(* Logix 5000 AddOnInstructionDefinition export Banner_Q5X_3000_Param_v4; software revision 33.00 *)

TYPE Banner_IOL_Port_v4 :   // UDT that has all of the data items necessary to communicate with a specific Port on a IO-Link Master
STRUCT
   Port_Controlled : INT;   // Each bit represents a port on an IO-Link Master. Set to 1 to tell AOI to control that port.
   Port_Activate : INT;   // Each bit represents a port on an IO-Link Master. When ON that port will process any commands in queue.
   Port_Read : INT;   // Each bit represents a port on an IO-Link Master. Used to determine when device AOI has requested a Read command.
   Port_Write : INT;   // Each bit represents a port on an IO-Link Master. Used to determine when device AOI has requested a Write command.
   Port_RW_Complete : INT;   // Each bit represents a port on an IO-Link Master. Tells device AOI that Read or Write request has been completed.
   Port_Device_Read : INT;
   Data_Transfer : SINT[190];   // Array to transfer data from IO-Master to device AOIs.
END_STRUCT
END_TYPE

TYPE Banner_Q5X_3000_RD_v4 :   // UDT that stores the Write Data for a Q5X TOF.
STRUCT
   Master_Cycle_Time : INT;
   Min_Cycle_Time : INT;
   M_Sequence_Capability : INT;
   IO_Link_Version_ID : INT;
   Process_Data_Input_Length : INT;
   Process_Data_Output_Length : INT;
   Combined_Vendor_ID : DINT;   // IO-Link Vendor ID
   Vendor_ID1 : INT;
   Vendor_ID2 : INT;
   Combined_Device_ID : DINT;   // IO-Link Device ID
   Device_ID1 : INT;
   Device_ID2 : INT;
   Device_ID3 : INT;
   Serial_Number : STRING;
   Teach_State : SINT;
   SP1_TP1 : SINT;
   SP1_TP2 : SINT;
   Measurement_1 : DINT;
   Excess_Gain : DINT;   // Amount of singla measured over the minimum threshold.
   Stability : SINT;
   Multiple_Peak_State : SINT;   // 0 = Multiple peaks not present, 1 = Multiple peaks present
   Emitter_Status : SINT;   // 0 = Active, 1 = Inactive
   Laser_Fault_Status : SINT;   // 0 = No Fault, 1 = Fault Present
   BDC1_Totalizer_Counts : DINT;
   Analog_Value : DINT;   // Output Analog value.
   Last_Taught_Temperature : DINT;   // Internal Temperature the last time device was taught.
   All_Time_Run_Time : DINT;   // Read only counter that tracks the total time sensor has been running since manufacture. Value in Hours.
   Display : STRING;   // Last Display information
   MDC_Lower_Limit : DINT;
   MDC_Upper_Limit : DINT;
   MDC_Unit : INT;
   MDC_Scale : SINT;
END_STRUCT
END_TYPE

TYPE Banner_Q5X_3000_v4 :   // All of the parameters for a Q5X Analog.
STRUCT
   Initial_Global_Read : BOOL;   // Determines if all of the IO-Link data has been read into the PLC yet
   Command : INT;   // Value placed in here will activate a read or write to a specifc IO-Link Index
   Read_Data : Banner_Q5X_3000_RD_v4;   // Read Only Data
   Write_Data : Banner_Q5X_3000_WD_v4;   // Write Data
   Archive : Banner_Q5X_3000_WD_v4;   // Archive Data
   Reset : BOOL;   // Resets AOI. This will force a complete parameter read of the sensor.
END_STRUCT
END_TYPE

TYPE Banner_Q5X_3000_WD_v4 :   // UDT that stores the Write Data for a Q5X Analog.
STRUCT
   System_Command : INT;   // See IODD file for list of commands that can be activated via the System Command interface
   Parameter_Access_Lock : SINT;   // Write access to all parameters is prohibited while value is 1. Only this parameter can be adjusted when value is 1.
   Data_Storage_Lock : SINT;   // Automatic data storage is disabled when this value is equal to 1. Read access is not affected.
   Local_Parameterization_Lock : SINT;   // Parameterization via local control elements on device is disabled.
   Local_User_Interface_Lock : SINT;   // Operation of local user interface is disabled.
   Teach_in_Channel : SINT;   // 0 = Default, 1 = BDC1, 2 = BDC2
   BDC1_Setpoint_1 : DINT;
   BDC1_Setpoint_2 : DINT;   // In FGS, defines the second switching point. Other modes do not use this parameter.
   BDC1_Switchpoint_Logic : INT;   // 0 = Light Operate, 1 = Dark Operate
   BDC1_Mode : INT;   // 1 = 1Pt BGS, 128 = 2Pt Static BGS, 129 = Dynamic BGS, 130 = 1Pt Window (FGS), 131 = Dual Teach
   BDC1_Hysteresis : INT;   // Hysteresis value for the switchpoint. A value of 0 will result in automatically calculated hysteresis
   Response_Speed : SINT;   // 0 = Speed 0, 1 = Speed 1, 2 = Speed 2, 3 = Speed 3
   Secondary_Output_Mode : SINT;   // 0 = Independent Output, 1 = Complementary Output, 2 = Pulse Frequency Output
   Zero_Reference_Location : SINT;   // 0 = Near, 1 = Far
   Shift_Zero_after_Teach : SINT;   // 0 = Off, 1 = On
   Display_Read : SINT;   // 0 = On, 1 = On Inverted, 2 = Off, 3 = Off Inverted
   Display_Units : SINT;   // 0 = Centimeters, 1 = Inches, 2 = Millimeters
   Pushbutton_Lockout : SINT;   // 0 = No Lockout, 1 = Pushbuttons Locked, 2 = Operator Lockout
   Output_Polarity : SINT;   // 0 = Default, 1 = PNP, 2 = NPN
   IOL_Filter_Time : INT;   // Time to average IOl process data measurement between updates
   Include_Binary : SINT;   // 0 = Include, 1 = Don't Include, 2= Measurement Device
   Measurement_1 : SINT;   // 0 = Disabled, 1 = Excess Gain, 2 = Excess Gain / 10, 3 = Channel 1 Dual Mode Percent
   Measurement_2 : SINT;   // 0 = Disabled, 1 = Distance Value, 2 = Displayed Distance, 3 = Channel 2 Dual Mode Percent
   BDC1_Delay_Mode : SINT;   // 0 = Disabled, 1 = On Off Delay, 2 = Oneshot, 3 = Totalizer
   BDC1_Delay_Timer_1 : DINT;   // 0 to 90000
   BDC1_Delay_Timer_2 : DINT;   // 0 to 90000
   BDC1_BGS_Teach_Offset : SINT;   // 0 = Auto, 1 = User Selected
   BDC1_FGS_Window_Size : SINT;   // 0 = Auto, 1 = User Selected
   BDC1_User_Teach_Offset : DINT;   // Mode must be FGS of BGS. Set the user defined offset. Can be positive or negative.
   BDC1_User_FGS_Window_Size : DINT;   // Mode must be FGS. Set the +/- window value.
   BDC1_Auto_Thresholding : SINT;   // 0 = On, 1 = Off, 2 = High Speed
   Resettable_Run_Time : DINT;
   AO1_Setpoint_SP1 : DINT;
   AO1_Setpoint_SP2 : DINT;
   AO1_Output_Type : SINT;   // 0 = 4-20mA, 1 = 0-10V
   AO1_Teach_Selection : SINT;   // 0 = 2-point, 1 = 1-point
   AO1_Slope : SINT;
   AO1_Loss_of_Signal : SINT;   // 0 = positive, 1 = negative
   AO1_Midpoint_Teach_Offset_Size : DINT;
   AO1_Trigger : SINT;   // 0 = Trigger Sample, 1 = Trigger Average, 2 = Trigger Max, 3 = Trigger Min, 4 = Trigger Range, 5 = Trigger Track Max, 6 = Trigger Track Min
   AO1_Average : SINT;
   All_Time_Run_Time_Event_Time : DINT;
   Resettable_Run_Time_Event_Time : DINT;
END_STRUCT
END_TYPE

ADD_ON_INSTRUCTION Banner_Q5X_3000_Param_v4   (* revision 4.1, vendor Banner Engineering *)
// AOI to read and write parameter data to an IO-Link Q5X 3000 Analog.
VAR_IN_OUT
   Q5X : Banner_Q5X_3000_v4; {required}
   Port_Data : Banner_IOL_Port_v4; {required}
END_VAR
VAR_INPUT
   Port : DINT; {required}
END_VAR
VAR
   Local_Control : DINT; {access None}
   Global_Read_Command_Value : INT; {access None}
   Global_Write_Command_Value : INT; {access None}
   Command_Being_Processed : BOOL; {access None}
   Update_Archive : BOOL; {access None}
   Index_Write_Inprocess : INT; {access None}
   Index_Write_Control : INT; {access None}
   Inprocess_Index : DINT; {access None}
END_VAR

ROUTINE Logic   (* ladder *)
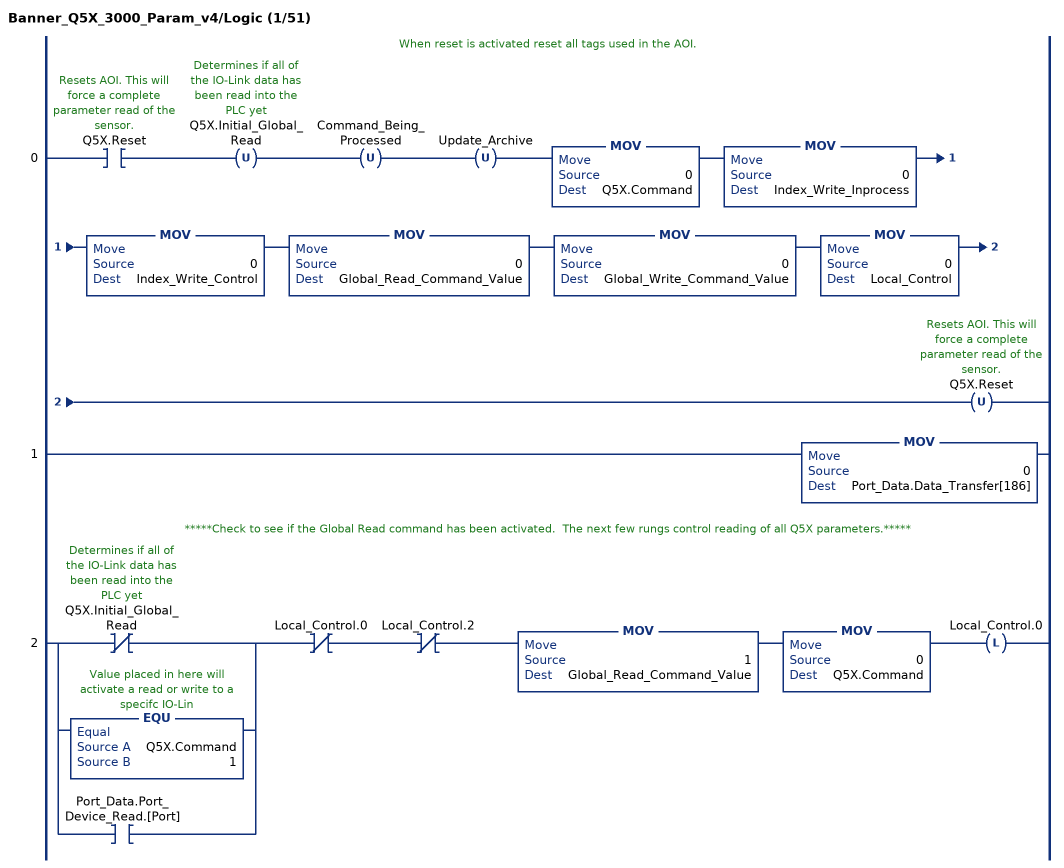
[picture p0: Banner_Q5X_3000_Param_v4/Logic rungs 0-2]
   // When reset is activated reset all tags used in the AOI.
   0: XIC(Q5X.Reset)OTU(Q5X.Initial_Global_Read)OTU(Command_Being_Processed)OTU(Update_Archive)MOV(0,Q5X.Command)MOV(0,Index_Write_Inprocess)MOV(0,Index_Write_Control)MOV(0,Global_Read_Command_Value)MOV(0,Global_Write_Command_Value)MOV(0,Local_Control)OTU(Q5X.Reset);
   1: MOV(0,Port_Data.Data_Transfer[186]);
   // *****Check to see if the Global Read command has been activated.  The next few rungs control reading of all Q5X parameters.*****
   2: [XIO(Q5X.Initial_Global_Read) ,EQU(Q5X.Command,1) ,XIC(Port_Data.Port_Device_Read.[Port]) ]XIO(Local_Control.0)XIO(Local_Control.2)MOV(1,Global_Read_Command_Value)MOV(0,Q5X.Command)OTL(Local_Control.0);
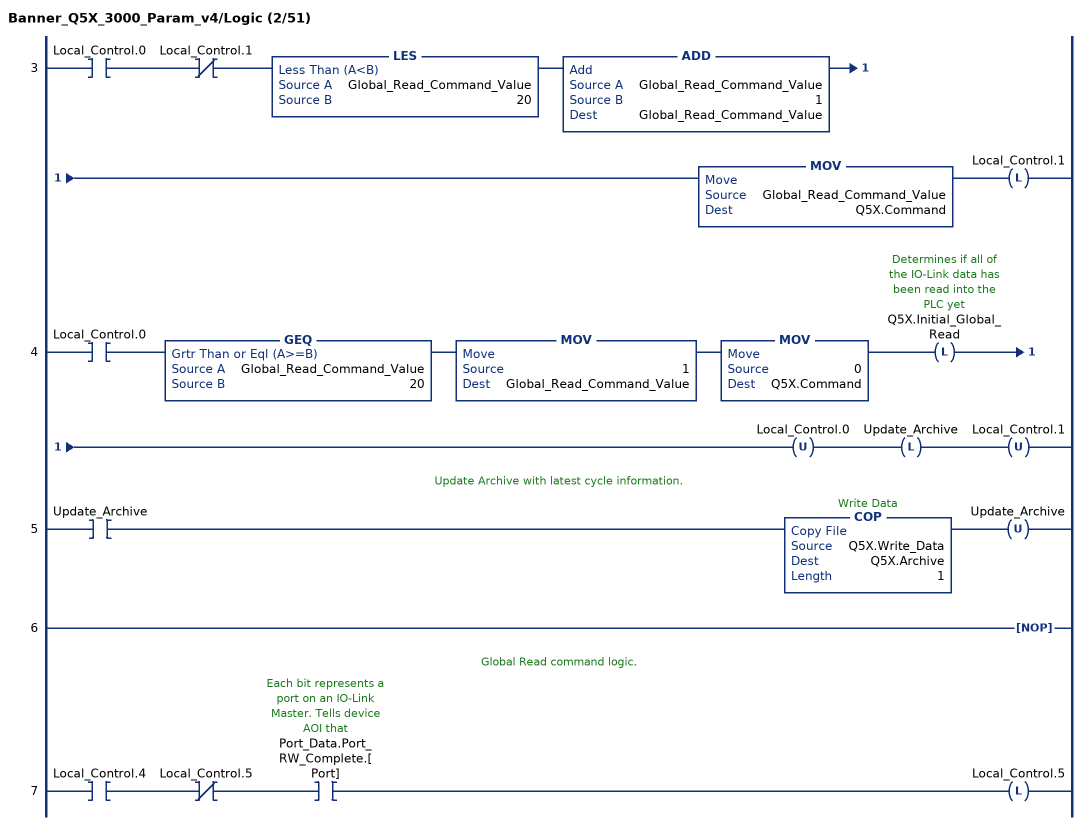
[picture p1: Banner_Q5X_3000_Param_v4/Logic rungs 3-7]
   3: XIC(Local_Control.0)XIO(Local_Control.1)LES(Global_Read_Command_Value,20)ADD(Global_Read_Command_Value,1,Global_Read_Command_Value)MOV(Global_Read_Command_Value,Q5X.Command)OTL(Local_Control.1);
   4: XIC(Local_Control.0)GEQ(Global_Read_Command_Value,20)MOV(1,Global_Read_Command_Value)MOV(0,Q5X.Command)OTL(Q5X.Initial_Global_Read)OTU(Local_Control.0)OTL(Update_Archive)OTU(Local_Control.1);
   // Update Archive with latest cycle information.
   5: XIC(Update_Archive)COP(Q5X.Write_Data,Q5X.Archive,1)OTU(Update_Archive);
   6: NOP();
   // Global Read command logic.
   7: XIC(Local_Control.4)XIO(Local_Control.5)XIC(Port_Data.Port_RW_Complete.[Port])OTL(Local_Control.5);
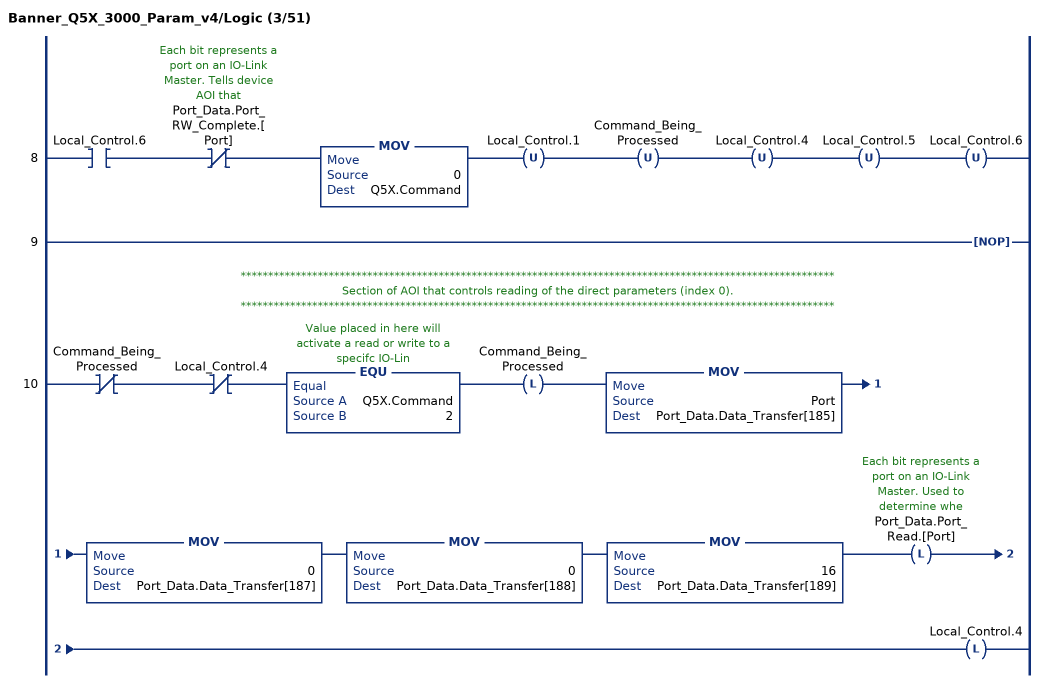
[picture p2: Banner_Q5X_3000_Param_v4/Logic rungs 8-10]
   8: XIC(Local_Control.6)XIO(Port_Data.Port_RW_Complete.[Port])MOV(0,Q5X.Command)OTU(Local_Control.1)OTU(Command_Being_Processed)OTU(Local_Control.4)OTU(Local_Control.5)OTU(Local_Control.6);
   9: NOP();
   // ************************************************************************************************************
   // Section of AOI that controls reading of the direct parameters (index 0).
   // ************************************************************************************************************
   10: XIO(Command_Being_Processed)XIO(Local_Control.4)EQU(Q5X.Command,2)OTL(Command_Being_Processed)MOV(Port,Port_Data.Data_Transfer[185])MOV(0,Port_Data.Data_Transfer[187])MOV(0,Port_Data.Data_Transfer[188])MOV(16,Port_Data.Data_Transfer[189])OTL(Port_Data.Port_Read.[Port])OTL(Local_Control.4);
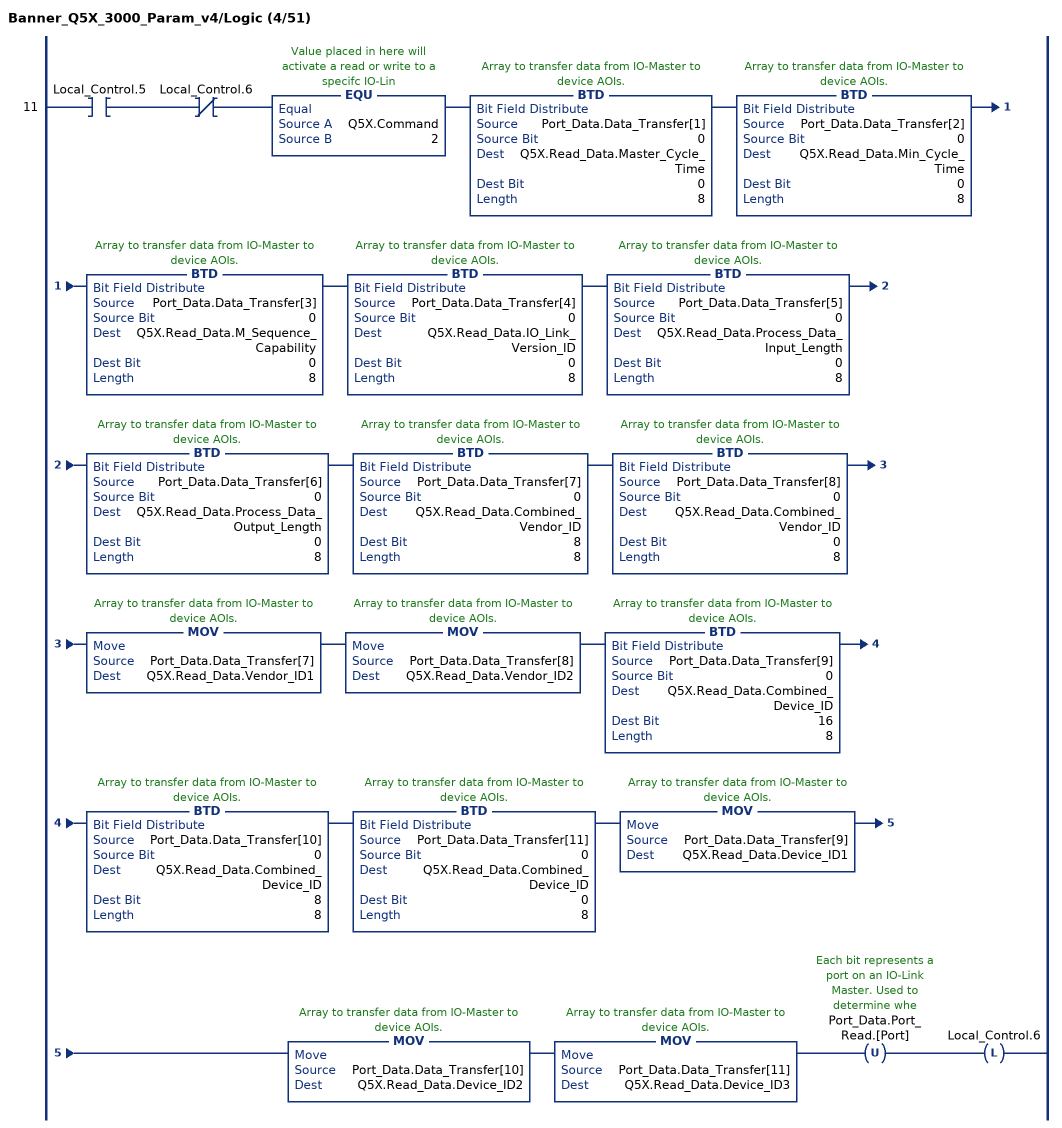
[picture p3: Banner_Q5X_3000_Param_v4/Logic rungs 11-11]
   11: XIC(Local_Control.5)XIO(Local_Control.6)EQU(Q5X.Command,2)BTD(Port_Data.Data_Transfer[1],0,Q5X.Read_Data.Master_Cycle_Time,0,8)BTD(Port_Data.Data_Transfer[2],0,Q5X.Read_Data.Min_Cycle_Time,0,8)BTD(Port_Data.Data_Transfer[3],0,Q5X.Read_Data.M_Sequence_Capability,0,8)BTD(Port_Data.Data_Transfer[4],0,Q5X.Read_Data.IO_Link_Version_ID,0,8)BTD(Port_Data.Data_Transfer[5],0,Q5X.Read_Data.Process_Data_Input_Length,0,8)BTD(Port_Data.Data_Transfer[6],0,Q5X.Read_Data.Process_Data_Output_Length,0,8)BTD(Port_Data.Data_Transfer[7],0,Q5X.Read_Data.Combined_Vendor_ID,8,8)BTD(Port_Data.Data_Transfer[8],0,Q5X.Read_Data.Combined_Vendor_ID,0,8)MOV(Port_Data.Data_Transfer[7],Q5X.Read_Data.Vendor_ID1)MOV(Port_Data.Data_Transfer[8],Q5X.Read_Data.Vendor_ID2)BTD(Port_Data.Data_Transfer[9],0,Q5X.Read_Data.Combined_Device_ID,16,8)BTD(Port_Data.Data_Transfer[10],0,Q5X.Read_Data.Combined_Device_ID,8,8)BTD(Port_Data.Data_Transfer[11],0,Q5X.Read_Data.Combined_Device_ID,0,8)MOV(Port_Data.Data_Transfer[9],Q5X.Read_Data.Device_ID1)MOV(Port_Data.Data_Transfer[10],Q5X.Read_Data.Device_ID2)MOV(Port_Data.Data_Transfer[11],Q5X.Read_Data.Device_ID3)OTU(Port_Data.Port_Read.[Port])OTL(Local_Control.6);
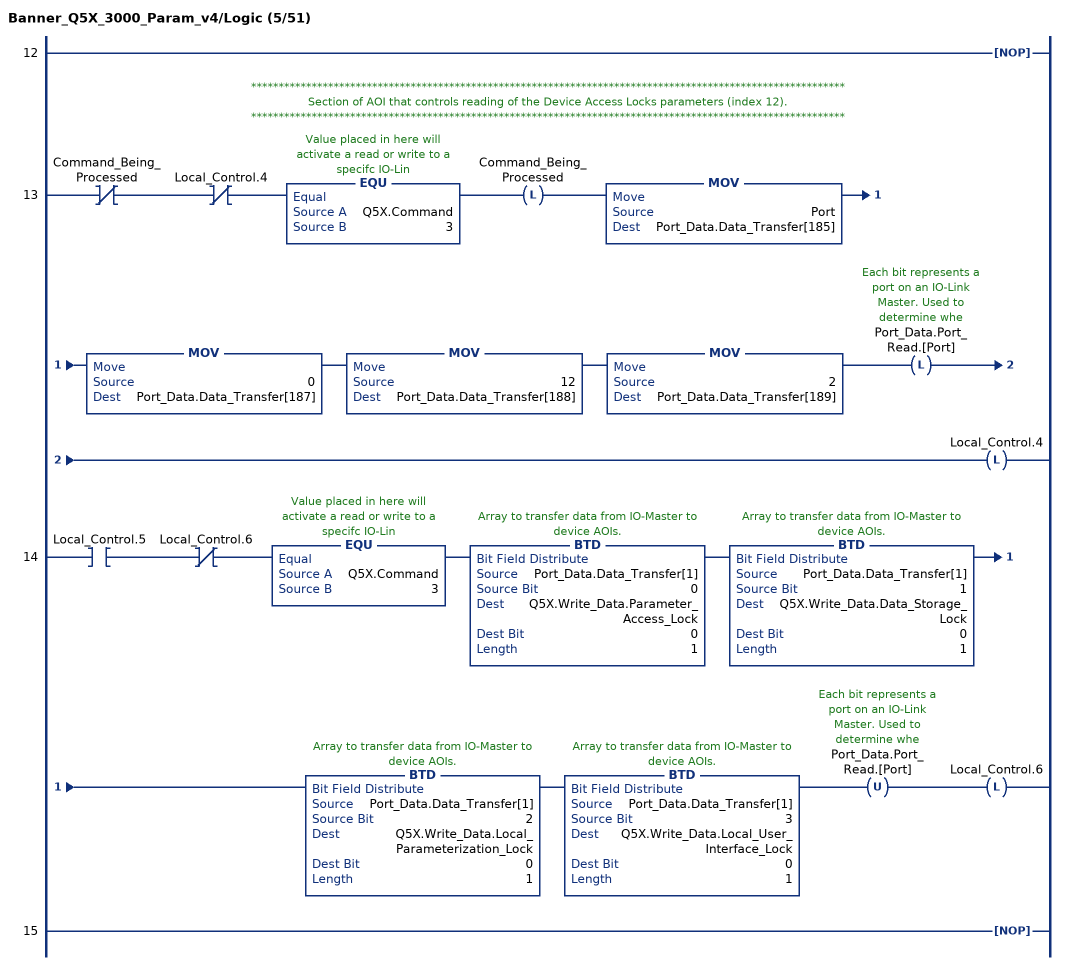
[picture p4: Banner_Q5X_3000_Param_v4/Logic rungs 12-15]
   12: NOP();
   // ************************************************************************************************************
   // Section of AOI that controls reading of the Device Access Locks parameters (index 12).
   // ************************************************************************************************************
   13: XIO(Command_Being_Processed)XIO(Local_Control.4)EQU(Q5X.Command,3)OTL(Command_Being_Processed)MOV(Port,Port_Data.Data_Transfer[185])MOV(0,Port_Data.Data_Transfer[187])MOV(12,Port_Data.Data_Transfer[188])MOV(2,Port_Data.Data_Transfer[189])OTL(Port_Data.Port_Read.[Port])OTL(Local_Control.4);
   14: XIC(Local_Control.5)XIO(Local_Control.6)EQU(Q5X.Command,3)BTD(Port_Data.Data_Transfer[1],0,Q5X.Write_Data.Parameter_Access_Lock,0,1)BTD(Port_Data.Data_Transfer[1],1,Q5X.Write_Data.Data_Storage_Lock,0,1)BTD(Port_Data.Data_Transfer[1],2,Q5X.Write_Data.Local_Parameterization_Lock,0,1)BTD(Port_Data.Data_Transfer[1],3,Q5X.Write_Data.Local_User_Interface_Lock,0,1)OTU(Port_Data.Port_Read.[Port])OTL(Local_Control.6);
   15: NOP();
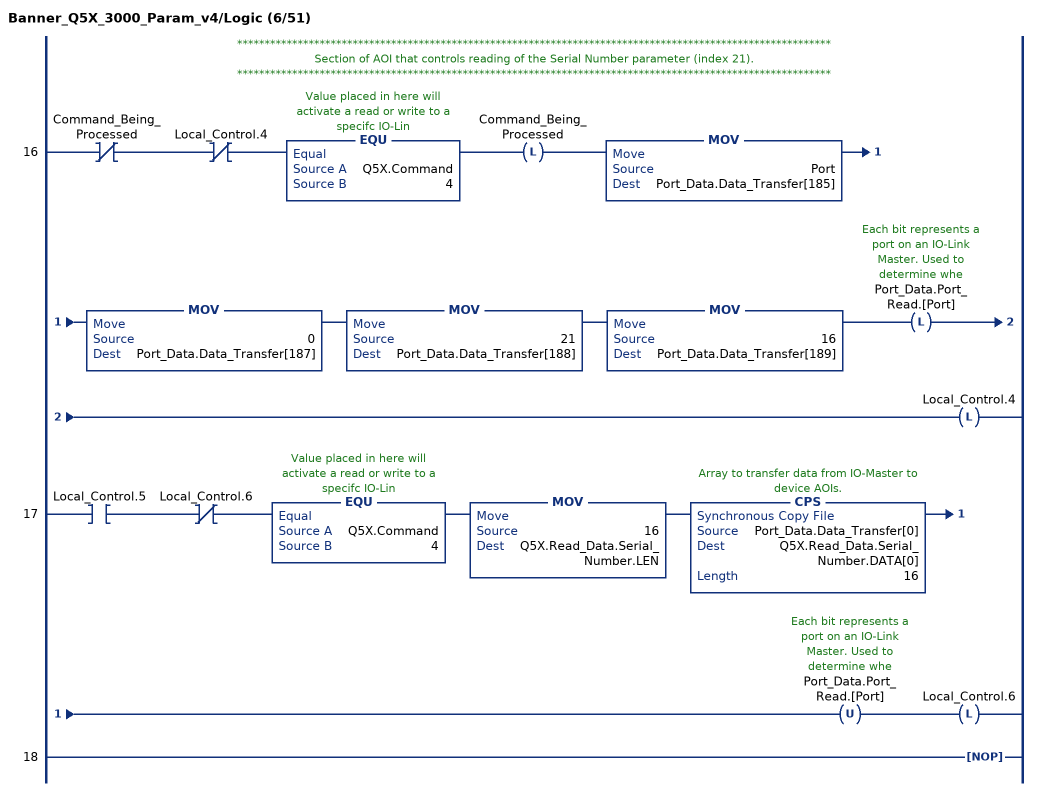
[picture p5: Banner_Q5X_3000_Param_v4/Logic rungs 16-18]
   // ************************************************************************************************************
   // Section of AOI that controls reading of the Serial Number parameter (index 21).
   // ************************************************************************************************************
   16: XIO(Command_Being_Processed)XIO(Local_Control.4)EQU(Q5X.Command,4)OTL(Command_Being_Processed)MOV(Port,Port_Data.Data_Transfer[185])MOV(0,Port_Data.Data_Transfer[187])MOV(21,Port_Data.Data_Transfer[188])MOV(16,Port_Data.Data_Transfer[189])OTL(Port_Data.Port_Read.[Port])OTL(Local_Control.4);
   17: XIC(Local_Control.5)XIO(Local_Control.6)EQU(Q5X.Command,4)MOV(16,Q5X.Read_Data.Serial_Number.LEN)CPS(Port_Data.Data_Transfer[0],Q5X.Read_Data.Serial_Number.DATA[0],16)OTU(Port_Data.Port_Read.[Port])OTL(Local_Control.6);
   18: NOP();
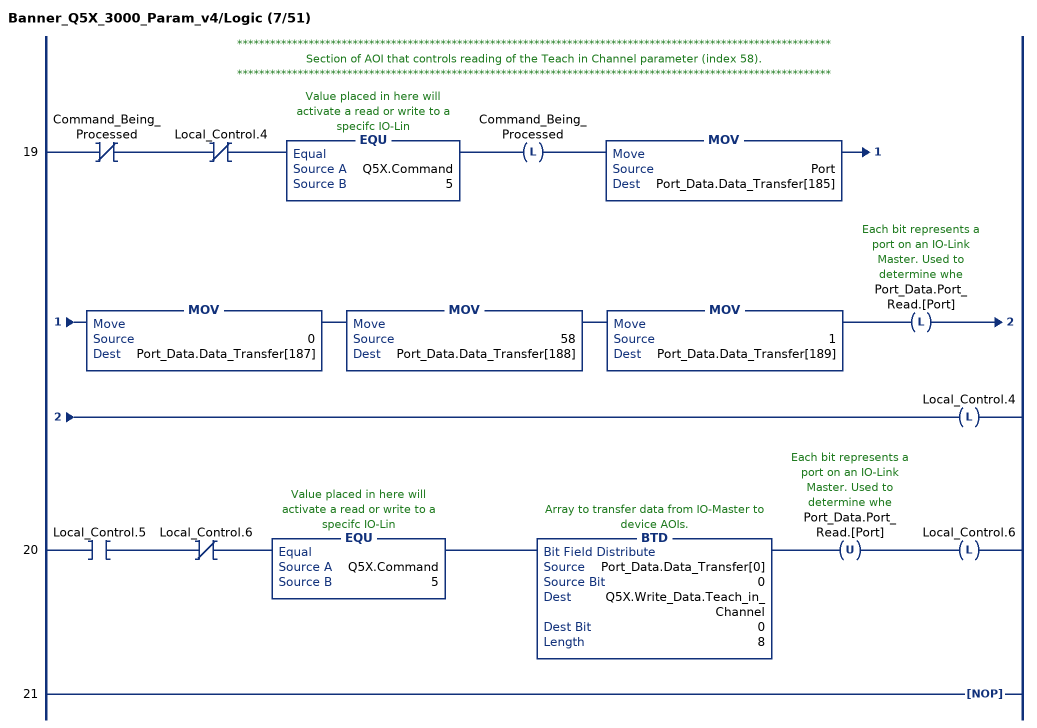
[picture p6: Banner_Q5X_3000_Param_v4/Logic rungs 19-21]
   // ************************************************************************************************************
   // Section of AOI that controls reading of the Teach in Channel parameter (index 58).
   // ************************************************************************************************************
   19: XIO(Command_Being_Processed)XIO(Local_Control.4)EQU(Q5X.Command,5)OTL(Command_Being_Processed)MOV(Port,Port_Data.Data_Transfer[185])MOV(0,Port_Data.Data_Transfer[187])MOV(58,Port_Data.Data_Transfer[188])MOV(1,Port_Data.Data_Transfer[189])OTL(Port_Data.Port_Read.[Port])OTL(Local_Control.4);
   20: XIC(Local_Control.5)XIO(Local_Control.6)EQU(Q5X.Command,5)BTD(Port_Data.Data_Transfer[0],0,Q5X.Write_Data.Teach_in_Channel,0,8)OTU(Port_Data.Port_Read.[Port])OTL(Local_Control.6);
   21: NOP();
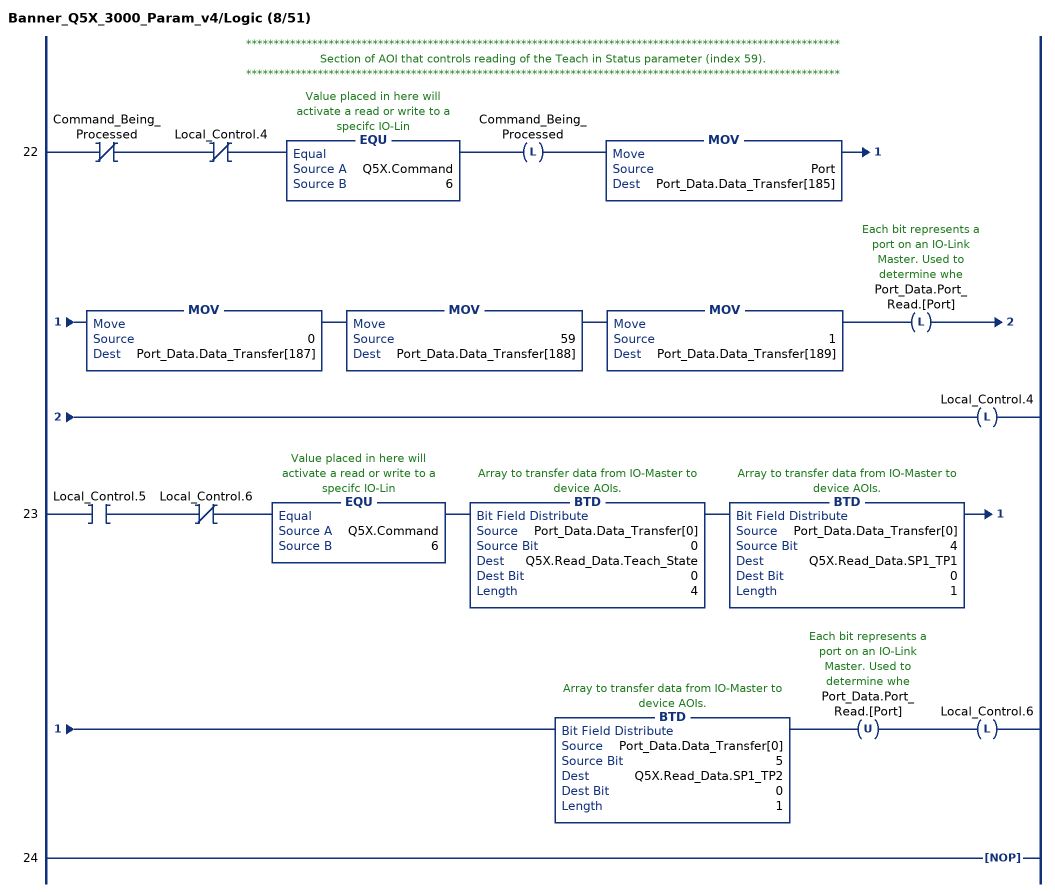
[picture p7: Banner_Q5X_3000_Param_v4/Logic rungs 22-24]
   // ************************************************************************************************************
   // Section of AOI that controls reading of the Teach in Status parameter (index 59).
   // ************************************************************************************************************
   22: XIO(Command_Being_Processed)XIO(Local_Control.4)EQU(Q5X.Command,6)OTL(Command_Being_Processed)MOV(Port,Port_Data.Data_Transfer[185])MOV(0,Port_Data.Data_Transfer[187])MOV(59,Port_Data.Data_Transfer[188])MOV(1,Port_Data.Data_Transfer[189])OTL(Port_Data.Port_Read.[Port])OTL(Local_Control.4);
   23: XIC(Local_Control.5)XIO(Local_Control.6)EQU(Q5X.Command,6)BTD(Port_Data.Data_Transfer[0],0,Q5X.Read_Data.Teach_State,0,4)BTD(Port_Data.Data_Transfer[0],4,Q5X.Read_Data.SP1_TP1,0,1)BTD(Port_Data.Data_Transfer[0],5,Q5X.Read_Data.SP1_TP2,0,1)OTU(Port_Data.Port_Read.[Port])OTL(Local_Control.6);
   24: NOP();
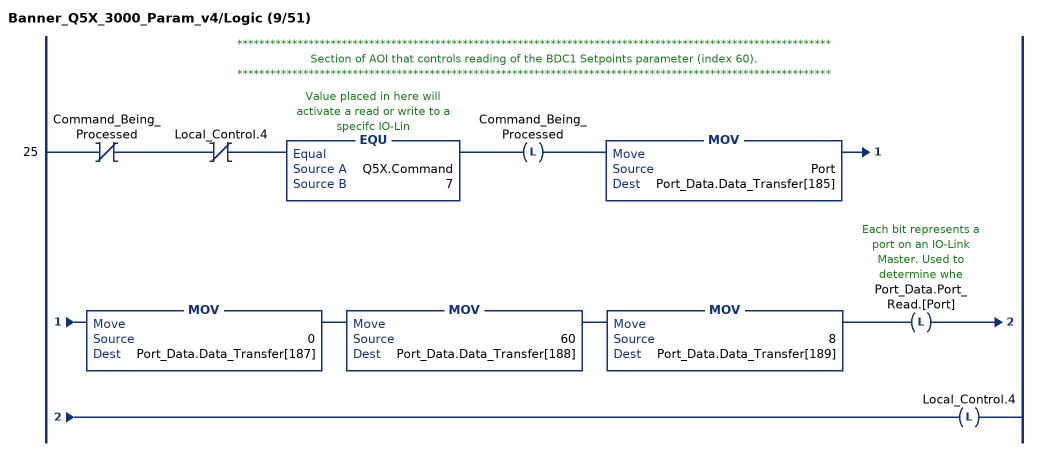
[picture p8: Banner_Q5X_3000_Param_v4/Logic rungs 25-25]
   // ************************************************************************************************************
   // Section of AOI that controls reading of the BDC1 Setpoints parameter (index 60).
   // ************************************************************************************************************
   25: XIO(Command_Being_Processed)XIO(Local_Control.4)EQU(Q5X.Command,7)OTL(Command_Being_Processed)MOV(Port,Port_Data.Data_Transfer[185])MOV(0,Port_Data.Data_Transfer[187])MOV(60,Port_Data.Data_Transfer[188])MOV(8,Port_Data.Data_Transfer[189])OTL(Port_Data.Port_Read.[Port])OTL(Local_Control.4);
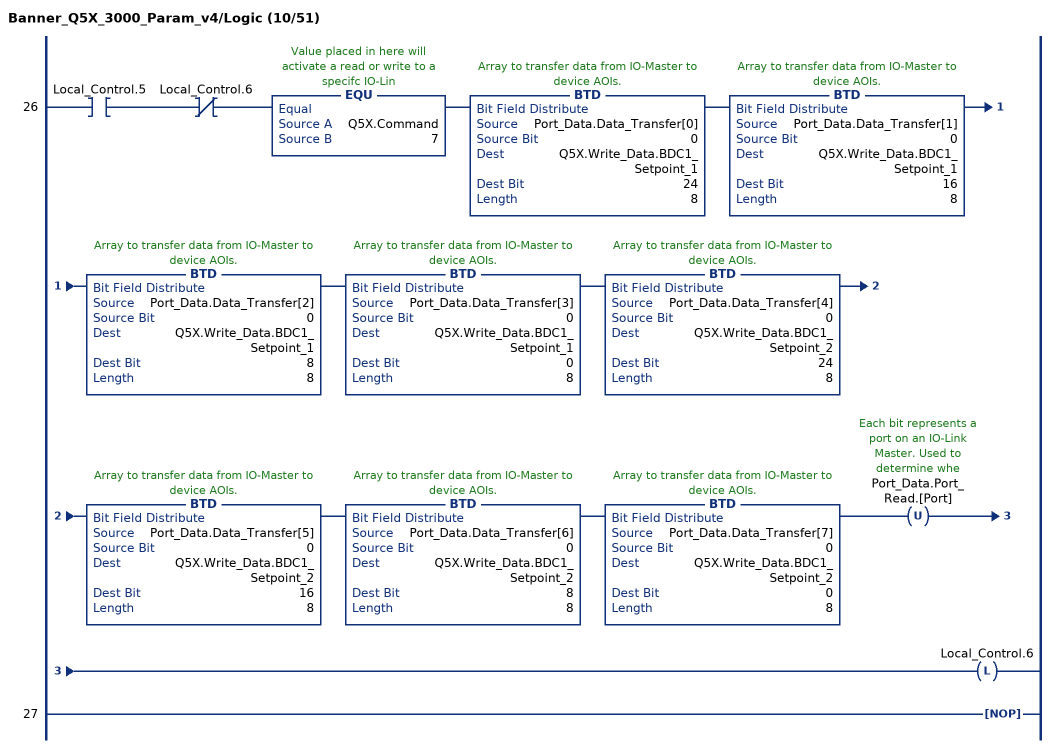
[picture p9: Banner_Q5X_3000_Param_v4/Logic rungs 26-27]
   26: XIC(Local_Control.5)XIO(Local_Control.6)EQU(Q5X.Command,7)BTD(Port_Data.Data_Transfer[0],0,Q5X.Write_Data.BDC1_Setpoint_1,24,8)BTD(Port_Data.Data_Transfer[1],0,Q5X.Write_Data.BDC1_Setpoint_1,16,8)BTD(Port_Data.Data_Transfer[2],0,Q5X.Write_Data.BDC1_Setpoint_1,8,8)BTD(Port_Data.Data_Transfer[3],0,Q5X.Write_Data.BDC1_Setpoint_1,0,8)BTD(Port_Data.Data_Transfer[4],0,Q5X.Write_Data.BDC1_Setpoint_2,24,8)BTD(Port_Data.Data_Transfer[5],0,Q5X.Write_Data.BDC1_Setpoint_2,16,8)BTD(Port_Data.Data_Transfer[6],0,Q5X.Write_Data.BDC1_Setpoint_2,8,8)BTD(Port_Data.Data_Transfer[7],0,Q5X.Write_Data.BDC1_Setpoint_2,0,8)OTU(Port_Data.Port_Read.[Port])OTL(Local_Control.6);
   27: NOP();
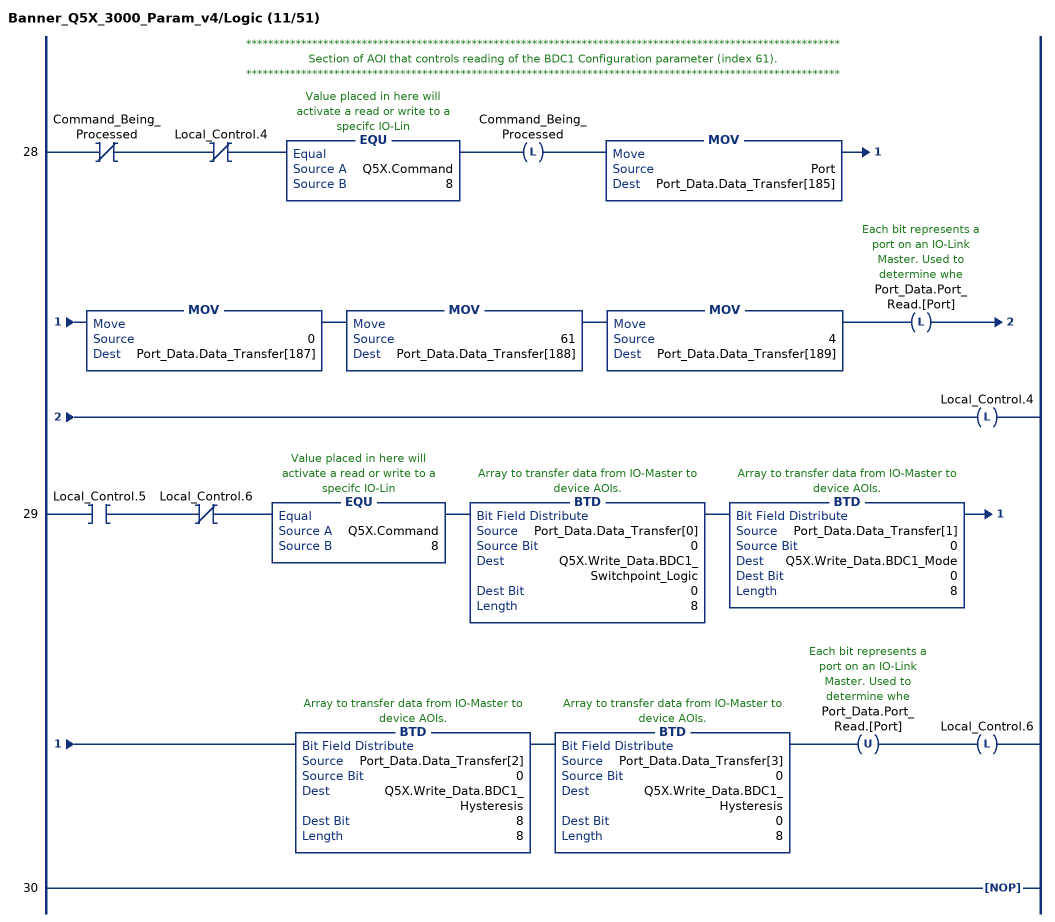
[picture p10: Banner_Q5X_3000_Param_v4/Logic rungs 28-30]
   // ************************************************************************************************************
   // Section of AOI that controls reading of the BDC1 Configuration parameter (index 61).
   // ************************************************************************************************************
   28: XIO(Command_Being_Processed)XIO(Local_Control.4)EQU(Q5X.Command,8)OTL(Command_Being_Processed)MOV(Port,Port_Data.Data_Transfer[185])MOV(0,Port_Data.Data_Transfer[187])MOV(61,Port_Data.Data_Transfer[188])MOV(4,Port_Data.Data_Transfer[189])OTL(Port_Data.Port_Read.[Port])OTL(Local_Control.4);
   29: XIC(Local_Control.5)XIO(Local_Control.6)EQU(Q5X.Command,8)BTD(Port_Data.Data_Transfer[0],0,Q5X.Write_Data.BDC1_Switchpoint_Logic,0,8)BTD(Port_Data.Data_Transfer[1],0,Q5X.Write_Data.BDC1_Mode,0,8)BTD(Port_Data.Data_Transfer[2],0,Q5X.Write_Data.BDC1_Hysteresis,8,8)BTD(Port_Data.Data_Transfer[3],0,Q5X.Write_Data.BDC1_Hysteresis,0,8)OTU(Port_Data.Port_Read.[Port])OTL(Local_Control.6);
   30: NOP();
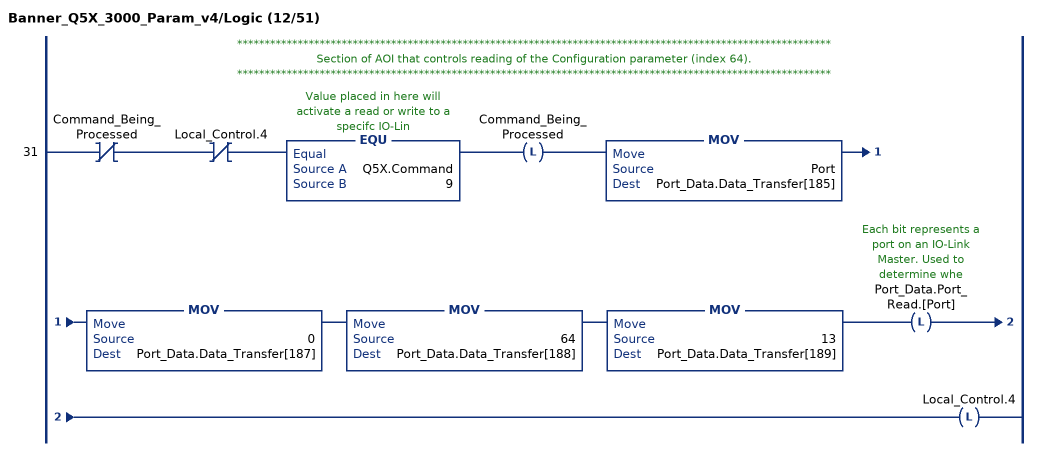
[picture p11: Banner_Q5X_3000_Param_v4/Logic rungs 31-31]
   // ************************************************************************************************************
   // Section of AOI that controls reading of the Configuration parameter (index 64).
   // ************************************************************************************************************
   31: XIO(Command_Being_Processed)XIO(Local_Control.4)EQU(Q5X.Command,9)OTL(Command_Being_Processed)MOV(Port,Port_Data.Data_Transfer[185])MOV(0,Port_Data.Data_Transfer[187])MOV(64,Port_Data.Data_Transfer[188])MOV(13,Port_Data.Data_Transfer[189])OTL(Port_Data.Port_Read.[Port])OTL(Local_Control.4);
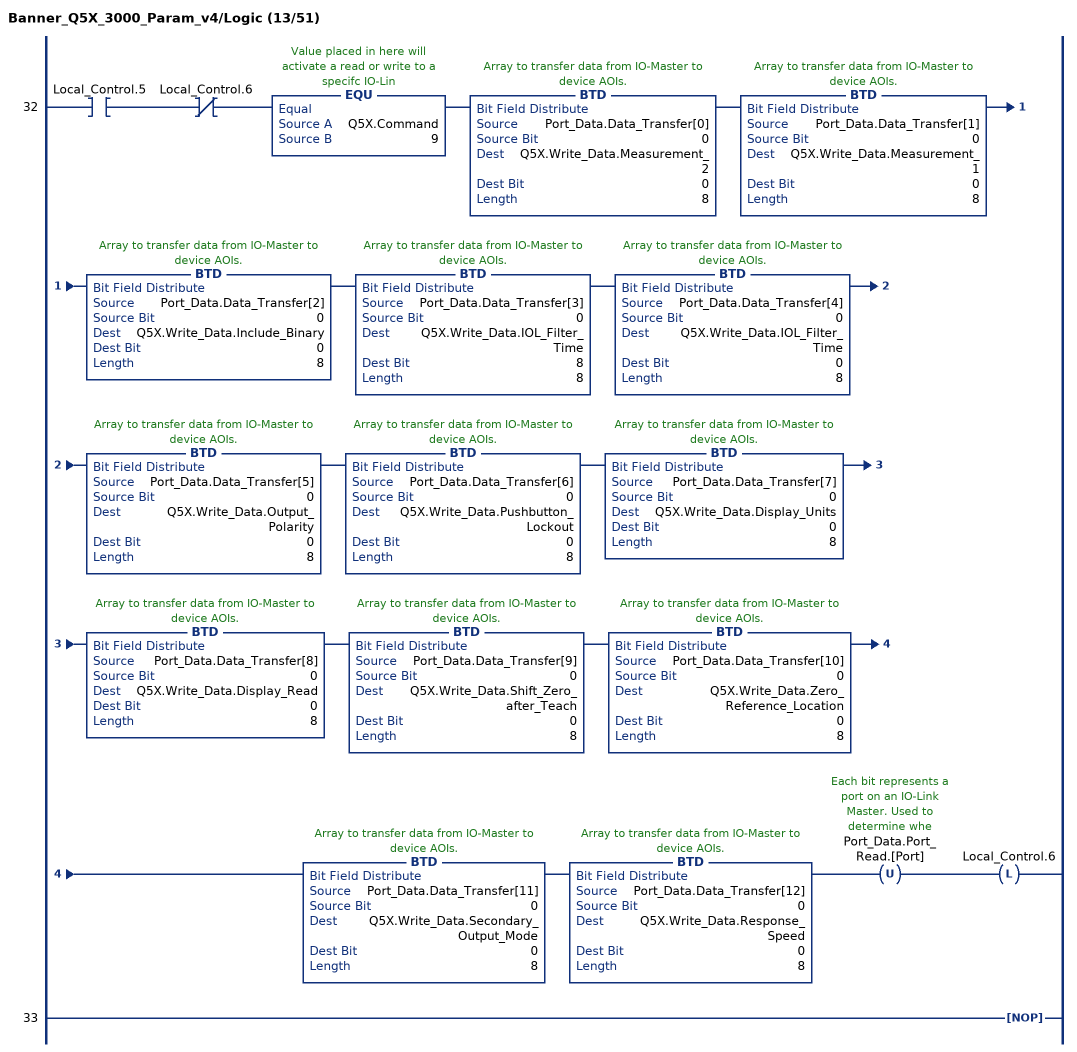
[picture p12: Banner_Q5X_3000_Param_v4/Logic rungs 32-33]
   32: XIC(Local_Control.5)XIO(Local_Control.6)EQU(Q5X.Command,9)BTD(Port_Data.Data_Transfer[0],0,Q5X.Write_Data.Measurement_2,0,8)BTD(Port_Data.Data_Transfer[1],0,Q5X.Write_Data.Measurement_1,0,8)BTD(Port_Data.Data_Transfer[2],0,Q5X.Write_Data.Include_Binary,0,8)BTD(Port_Data.Data_Transfer[3],0,Q5X.Write_Data.IOL_Filter_Time,8,8)BTD(Port_Data.Data_Transfer[4],0,Q5X.Write_Data.IOL_Filter_Time,0,8)BTD(Port_Data.Data_Transfer[5],0,Q5X.Write_Data.Output_Polarity,0,8)BTD(Port_Data.Data_Transfer[6],0,Q5X.Write_Data.Pushbutton_Lockout,0,8)BTD(Port_Data.Data_Transfer[7],0,Q5X.Write_Data.Display_Units,0,8)BTD(Port_Data.Data_Transfer[8],0,Q5X.Write_Data.Display_Read,0,8)BTD(Port_Data.Data_Transfer[9],0,Q5X.Write_Data.Shift_Zero_after_Teach,0,8)BTD(Port_Data.Data_Transfer[10],0,Q5X.Write_Data.Zero_Reference_Location,0,8)BTD(Port_Data.Data_Transfer[11],0,Q5X.Write_Data.Secondary_Output_Mode,0,8)BTD(Port_Data.Data_Transfer[12],0,Q5X.Write_Data.Response_Speed,0,8)OTU(Port_Data.Port_Read.[Port])OTL(Local_Control.6);
   33: NOP();
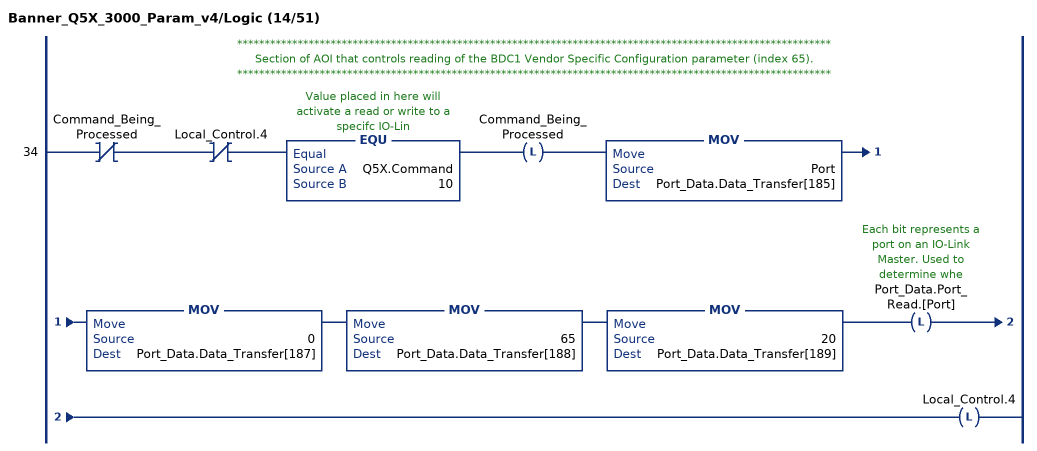
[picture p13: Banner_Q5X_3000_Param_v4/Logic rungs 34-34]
   // ************************************************************************************************************
   // Section of AOI that controls reading of the BDC1 Vendor Specific Configuration parameter (index 65).
   // ************************************************************************************************************
   34: XIO(Command_Being_Processed)XIO(Local_Control.4)EQU(Q5X.Command,10)OTL(Command_Being_Processed)MOV(Port,Port_Data.Data_Transfer[185])MOV(0,Port_Data.Data_Transfer[187])MOV(65,Port_Data.Data_Transfer[188])MOV(20,Port_Data.Data_Transfer[189])OTL(Port_Data.Port_Read.[Port])OTL(Local_Control.4);
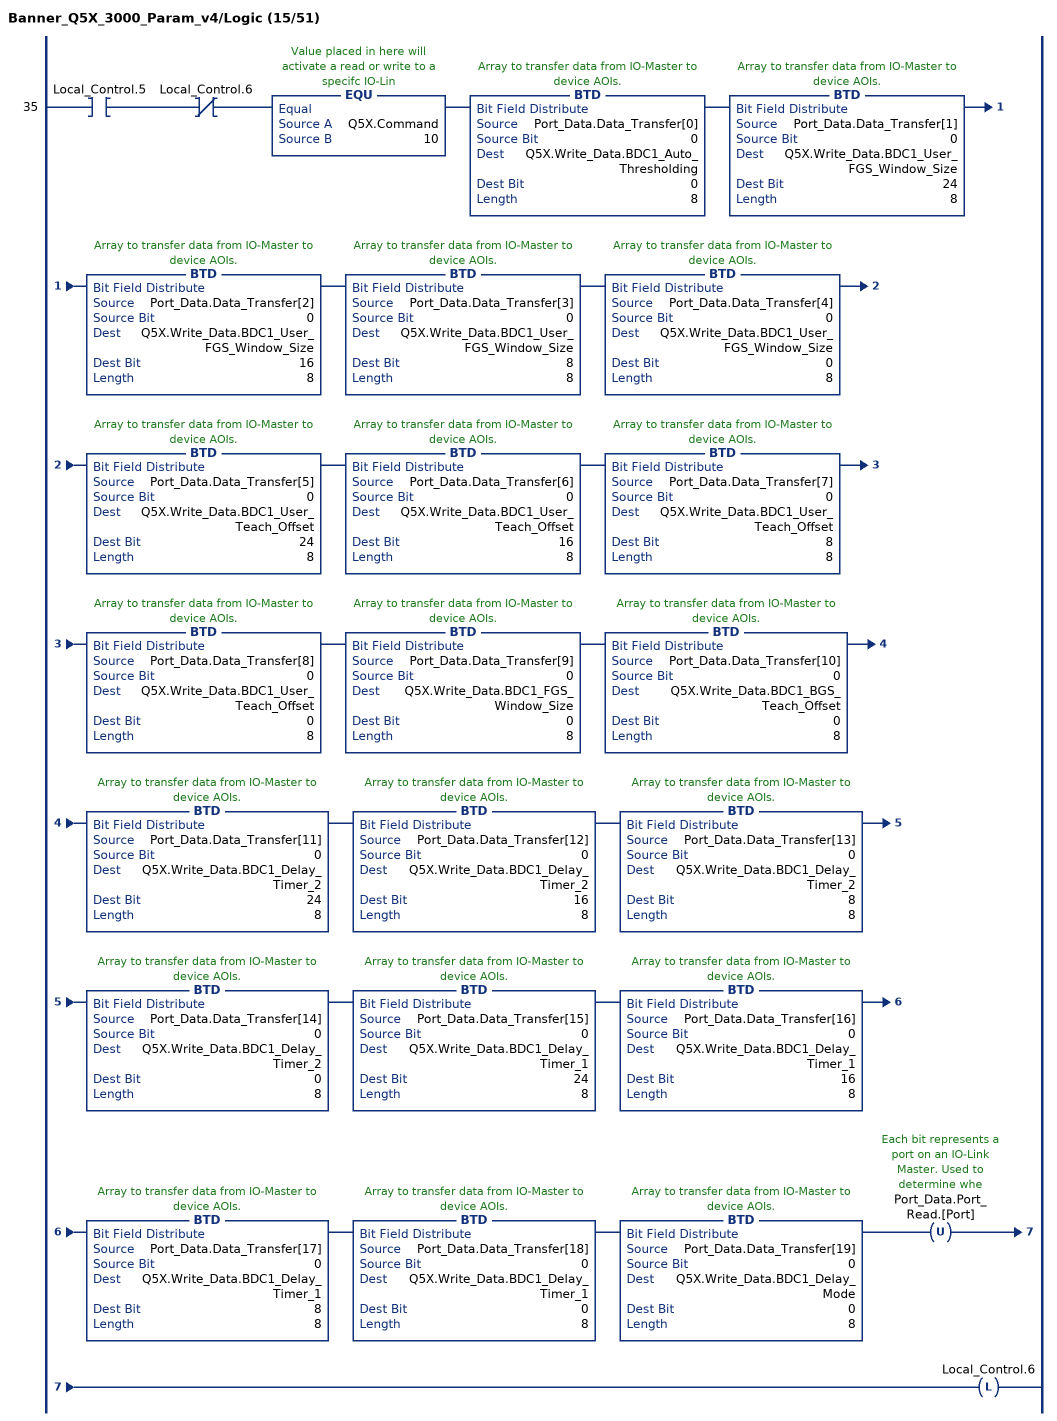
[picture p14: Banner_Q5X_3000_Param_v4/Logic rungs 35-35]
   35: XIC(Local_Control.5)XIO(Local_Control.6)EQU(Q5X.Command,10)BTD(Port_Data.Data_Transfer[0],0,Q5X.Write_Data.BDC1_Auto_Thresholding,0,8)BTD(Port_Data.Data_Transfer[1],0,Q5X.Write_Data.BDC1_User_FGS_Window_Size,24,8)BTD(Port_Data.Data_Transfer[2],0,Q5X.Write_Data.BDC1_User_FGS_Window_Size,16,8)BTD(Port_Data.Data_Transfer[3],0,Q5X.Write_Data.BDC1_User_FGS_Window_Size,8,8)BTD(Port_Data.Data_Transfer[4],0,Q5X.Write_Data.BDC1_User_FGS_Window_Size,0,8)BTD(Port_Data.Data_Transfer[5],0,Q5X.Write_Data.BDC1_User_Teach_Offset,24,8)BTD(Port_Data.Data_Transfer[6],0,Q5X.Write_Data.BDC1_User_Teach_Offset,16,8)BTD(Port_Data.Data_Transfer[7],0,Q5X.Write_Data.BDC1_User_Teach_Offset,8,8)BTD(Port_Data.Data_Transfer[8],0,Q5X.Write_Data.BDC1_User_Teach_Offset,0,8)BTD(Port_Data.Data_Transfer[9],0,Q5X.Write_Data.BDC1_FGS_Window_Size,0,8)BTD(Port_Data.Data_Transfer[10],0,Q5X.Write_Data.BDC1_BGS_Teach_Offset,0,8)BTD(Port_Data.Data_Transfer[11],0,Q5X.Write_Data.BDC1_Delay_Timer_2,24,8)BTD(Port_Data.Data_Transfer[12],0,Q5X.Write_Data.BDC1_Delay_Timer_2,16,8)BTD(Port_Data.Data_Transfer[13],0,Q5X.Write_Data.BDC1_Delay_Timer_2,8,8)BTD(Port_Data.Data_Transfer[14],0,Q5X.Write_Data.BDC1_Delay_Timer_2,0,8)BTD(Port_Data.Data_Transfer[15],0,Q5X.Write_Data.BDC1_Delay_Timer_1,24,8)BTD(Port_Data.Data_Transfer[16],0,Q5X.Write_Data.BDC1_Delay_Timer_1,16,8)BTD(Port_Data.Data_Transfer[17],0,Q5X.Write_Data.BDC1_Delay_Timer_1,8,8)BTD(Port_Data.Data_Transfer[18],0,Q5X.Write_Data.BDC1_Delay_Timer_1,0,8)BTD(Port_Data.Data_Transfer[19],0,Q5X.Write_Data.BDC1_Delay_Mode,0,8)OTU(Port_Data.Port_Read.[Port])OTL(Local_Control.6);
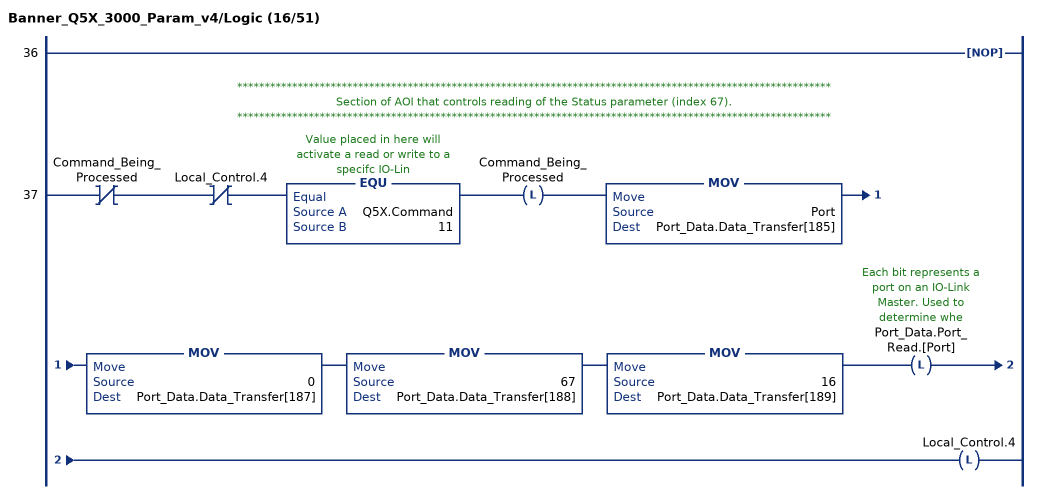
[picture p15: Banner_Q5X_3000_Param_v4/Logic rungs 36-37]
   36: NOP();
   // ************************************************************************************************************
   // Section of AOI that controls reading of the Status parameter (index 67).
   // ************************************************************************************************************
   37: XIO(Command_Being_Processed)XIO(Local_Control.4)EQU(Q5X.Command,11)OTL(Command_Being_Processed)MOV(Port,Port_Data.Data_Transfer[185])MOV(0,Port_Data.Data_Transfer[187])MOV(67,Port_Data.Data_Transfer[188])MOV(16,Port_Data.Data_Transfer[189])OTL(Port_Data.Port_Read.[Port])OTL(Local_Control.4);
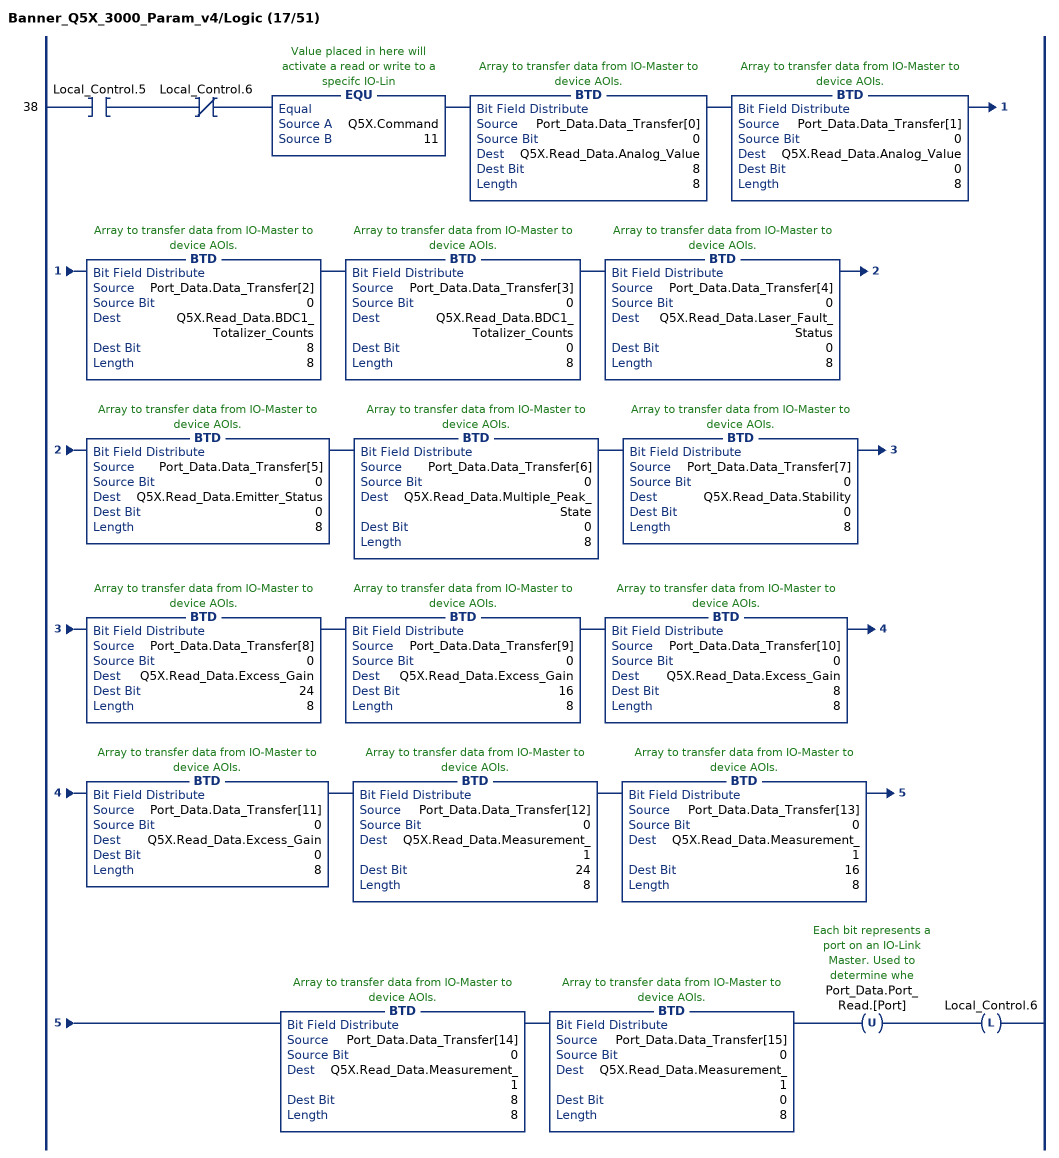
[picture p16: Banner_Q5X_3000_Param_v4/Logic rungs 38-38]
   38: XIC(Local_Control.5)XIO(Local_Control.6)EQU(Q5X.Command,11)BTD(Port_Data.Data_Transfer[0],0,Q5X.Read_Data.Analog_Value,8,8)BTD(Port_Data.Data_Transfer[1],0,Q5X.Read_Data.Analog_Value,0,8)BTD(Port_Data.Data_Transfer[2],0,Q5X.Read_Data.BDC1_Totalizer_Counts,8,8)BTD(Port_Data.Data_Transfer[3],0,Q5X.Read_Data.BDC1_Totalizer_Counts,0,8)BTD(Port_Data.Data_Transfer[4],0,Q5X.Read_Data.Laser_Fault_Status,0,8)BTD(Port_Data.Data_Transfer[5],0,Q5X.Read_Data.Emitter_Status,0,8)BTD(Port_Data.Data_Transfer[6],0,Q5X.Read_Data.Multiple_Peak_State,0,8)BTD(Port_Data.Data_Transfer[7],0,Q5X.Read_Data.Stability,0,8)BTD(Port_Data.Data_Transfer[8],0,Q5X.Read_Data.Excess_Gain,24,8)BTD(Port_Data.Data_Transfer[9],0,Q5X.Read_Data.Excess_Gain,16,8)BTD(Port_Data.Data_Transfer[10],0,Q5X.Read_Data.Excess_Gain,8,8)BTD(Port_Data.Data_Transfer[11],0,Q5X.Read_Data.Excess_Gain,0,8)BTD(Port_Data.Data_Transfer[12],0,Q5X.Read_Data.Measurement_1,24,8)BTD(Port_Data.Data_Transfer[13],0,Q5X.Read_Data.Measurement_1,16,8)BTD(Port_Data.Data_Transfer[14],0,Q5X.Read_Data.Measurement_1,8,8)BTD(Port_Data.Data_Transfer[15],0,Q5X.Read_Data.Measurement_1,0,8)OTU(Port_Data.Port_Read.[Port])OTL(Local_Control.6);
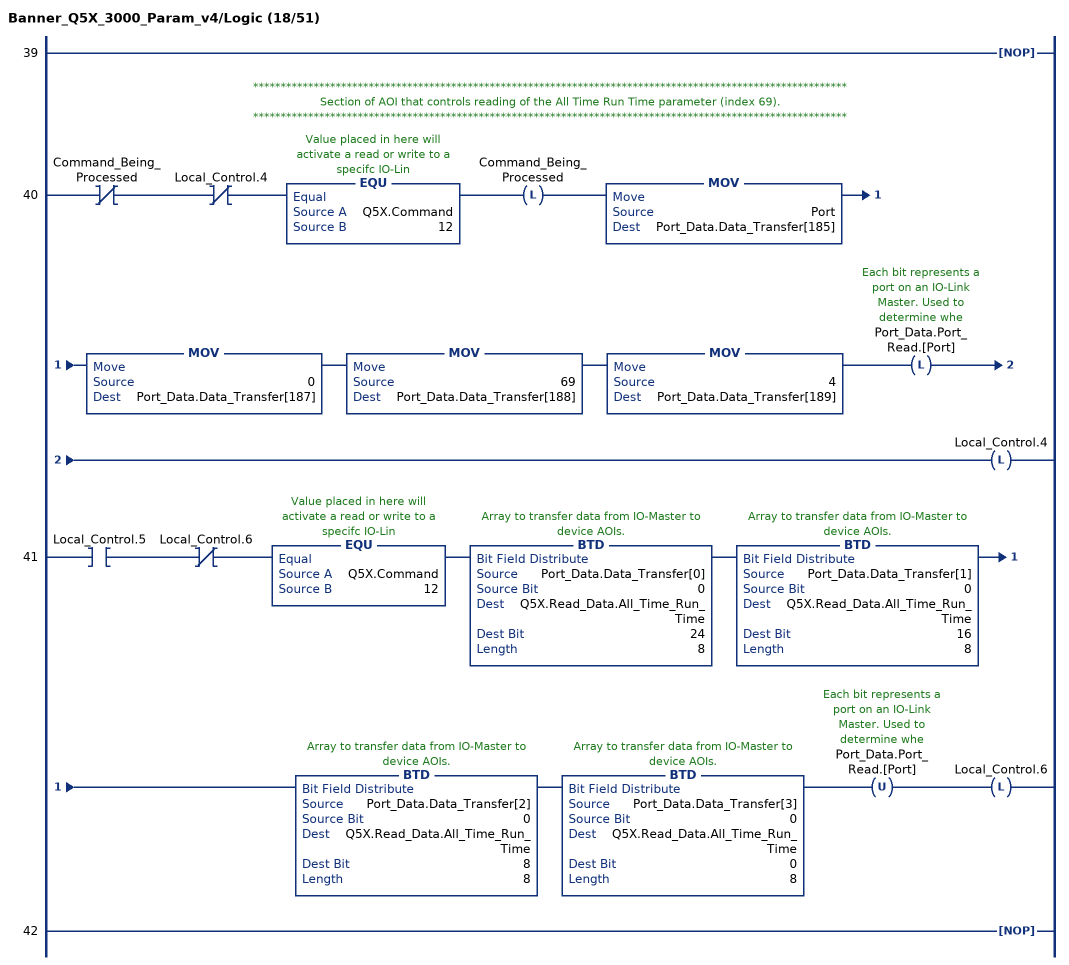
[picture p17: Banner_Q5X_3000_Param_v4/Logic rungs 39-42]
   39: NOP();
   // ************************************************************************************************************
   // Section of AOI that controls reading of the All Time Run Time parameter (index 69).
   // ************************************************************************************************************
   40: XIO(Command_Being_Processed)XIO(Local_Control.4)EQU(Q5X.Command,12)OTL(Command_Being_Processed)MOV(Port,Port_Data.Data_Transfer[185])MOV(0,Port_Data.Data_Transfer[187])MOV(69,Port_Data.Data_Transfer[188])MOV(4,Port_Data.Data_Transfer[189])OTL(Port_Data.Port_Read.[Port])OTL(Local_Control.4);
   41: XIC(Local_Control.5)XIO(Local_Control.6)EQU(Q5X.Command,12)BTD(Port_Data.Data_Transfer[0],0,Q5X.Read_Data.All_Time_Run_Time,24,8)BTD(Port_Data.Data_Transfer[1],0,Q5X.Read_Data.All_Time_Run_Time,16,8)BTD(Port_Data.Data_Transfer[2],0,Q5X.Read_Data.All_Time_Run_Time,8,8)BTD(Port_Data.Data_Transfer[3],0,Q5X.Read_Data.All_Time_Run_Time,0,8)OTU(Port_Data.Port_Read.[Port])OTL(Local_Control.6);
   42: NOP();
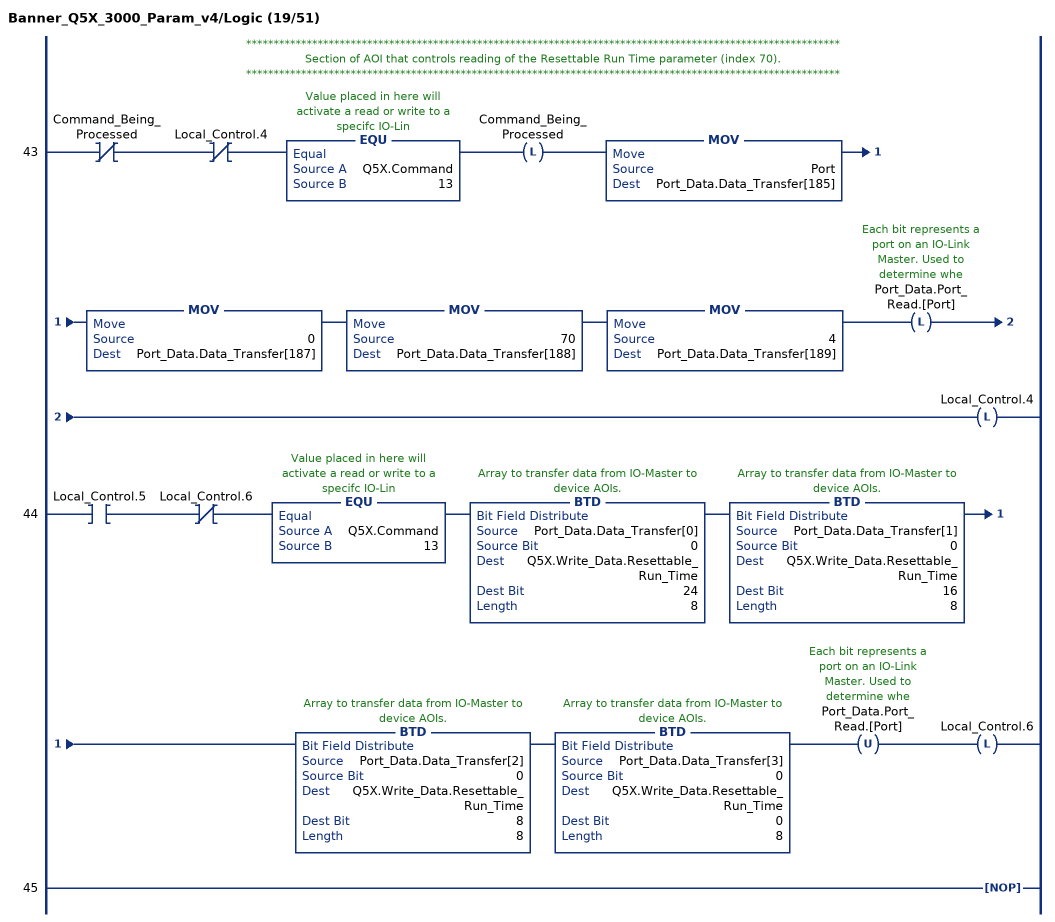
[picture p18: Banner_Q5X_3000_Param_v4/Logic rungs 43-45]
   // ************************************************************************************************************
   // Section of AOI that controls reading of the Resettable Run Time parameter (index 70).
   // ************************************************************************************************************
   43: XIO(Command_Being_Processed)XIO(Local_Control.4)EQU(Q5X.Command,13)OTL(Command_Being_Processed)MOV(Port,Port_Data.Data_Transfer[185])MOV(0,Port_Data.Data_Transfer[187])MOV(70,Port_Data.Data_Transfer[188])MOV(4,Port_Data.Data_Transfer[189])OTL(Port_Data.Port_Read.[Port])OTL(Local_Control.4);
   44: XIC(Local_Control.5)XIO(Local_Control.6)EQU(Q5X.Command,13)BTD(Port_Data.Data_Transfer[0],0,Q5X.Write_Data.Resettable_Run_Time,24,8)BTD(Port_Data.Data_Transfer[1],0,Q5X.Write_Data.Resettable_Run_Time,16,8)BTD(Port_Data.Data_Transfer[2],0,Q5X.Write_Data.Resettable_Run_Time,8,8)BTD(Port_Data.Data_Transfer[3],0,Q5X.Write_Data.Resettable_Run_Time,0,8)OTU(Port_Data.Port_Read.[Port])OTL(Local_Control.6);
   45: NOP();
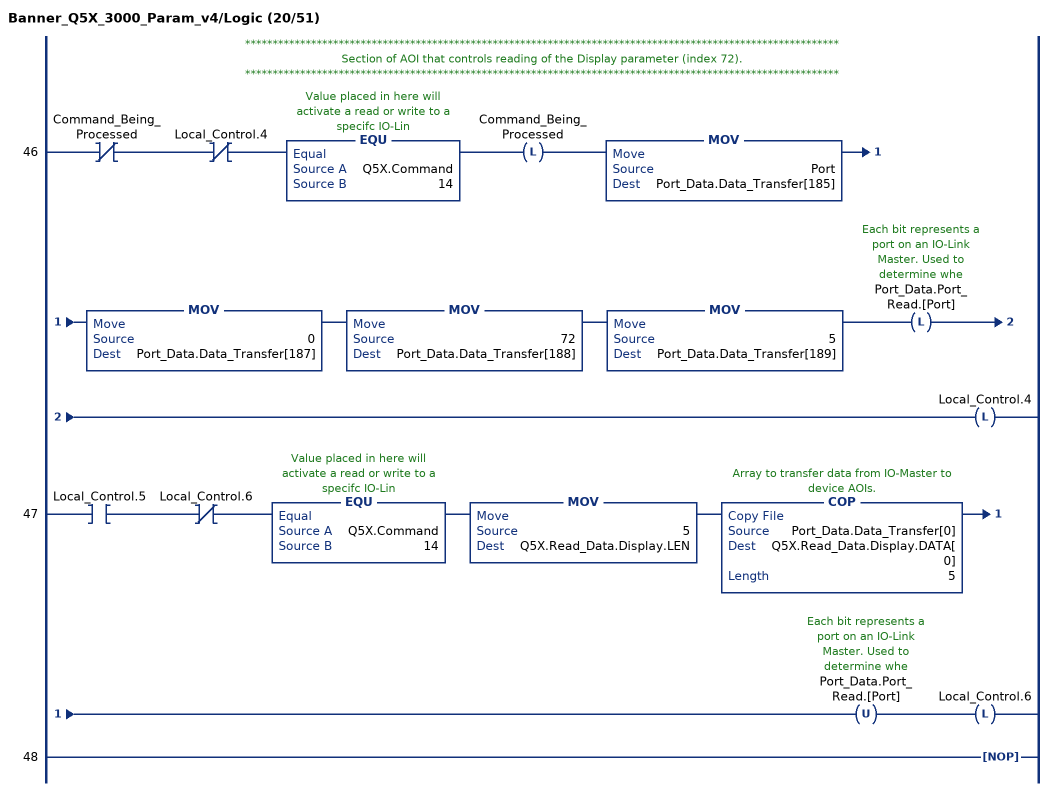
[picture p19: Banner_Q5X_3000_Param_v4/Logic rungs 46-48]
   // ************************************************************************************************************
   // Section of AOI that controls reading of the Display parameter (index 72).
   // ************************************************************************************************************
   46: XIO(Command_Being_Processed)XIO(Local_Control.4)EQU(Q5X.Command,14)OTL(Command_Being_Processed)MOV(Port,Port_Data.Data_Transfer[185])MOV(0,Port_Data.Data_Transfer[187])MOV(72,Port_Data.Data_Transfer[188])MOV(5,Port_Data.Data_Transfer[189])OTL(Port_Data.Port_Read.[Port])OTL(Local_Control.4);
   47: XIC(Local_Control.5)XIO(Local_Control.6)EQU(Q5X.Command,14)MOV(5,Q5X.Read_Data.Display.LEN)COP(Port_Data.Data_Transfer[0],Q5X.Read_Data.Display.DATA[0],5)OTU(Port_Data.Port_Read.[Port])OTL(Local_Control.6);
   48: NOP();
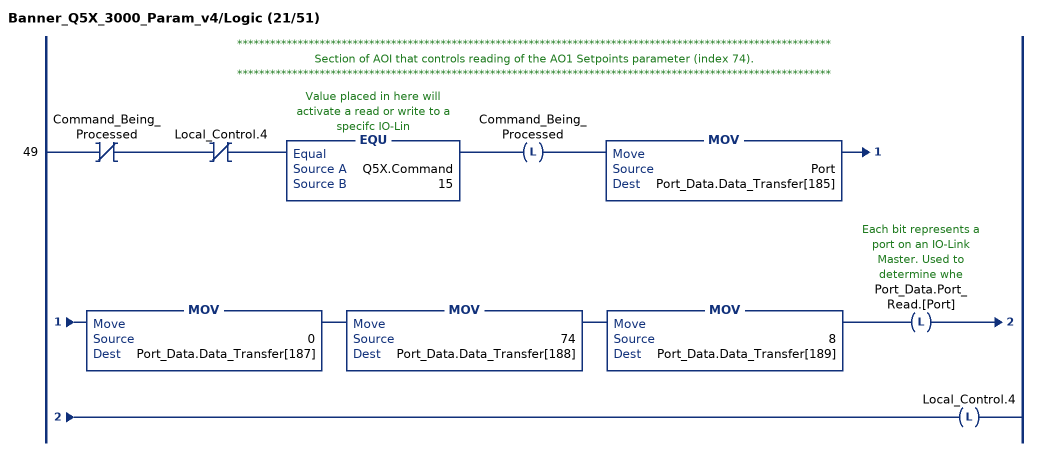
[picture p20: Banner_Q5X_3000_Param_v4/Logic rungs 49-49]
   // ************************************************************************************************************
   // Section of AOI that controls reading of the AO1 Setpoints parameter (index 74).
   // ************************************************************************************************************
   49: XIO(Command_Being_Processed)XIO(Local_Control.4)EQU(Q5X.Command,15)OTL(Command_Being_Processed)MOV(Port,Port_Data.Data_Transfer[185])MOV(0,Port_Data.Data_Transfer[187])MOV(74,Port_Data.Data_Transfer[188])MOV(8,Port_Data.Data_Transfer[189])OTL(Port_Data.Port_Read.[Port])OTL(Local_Control.4);
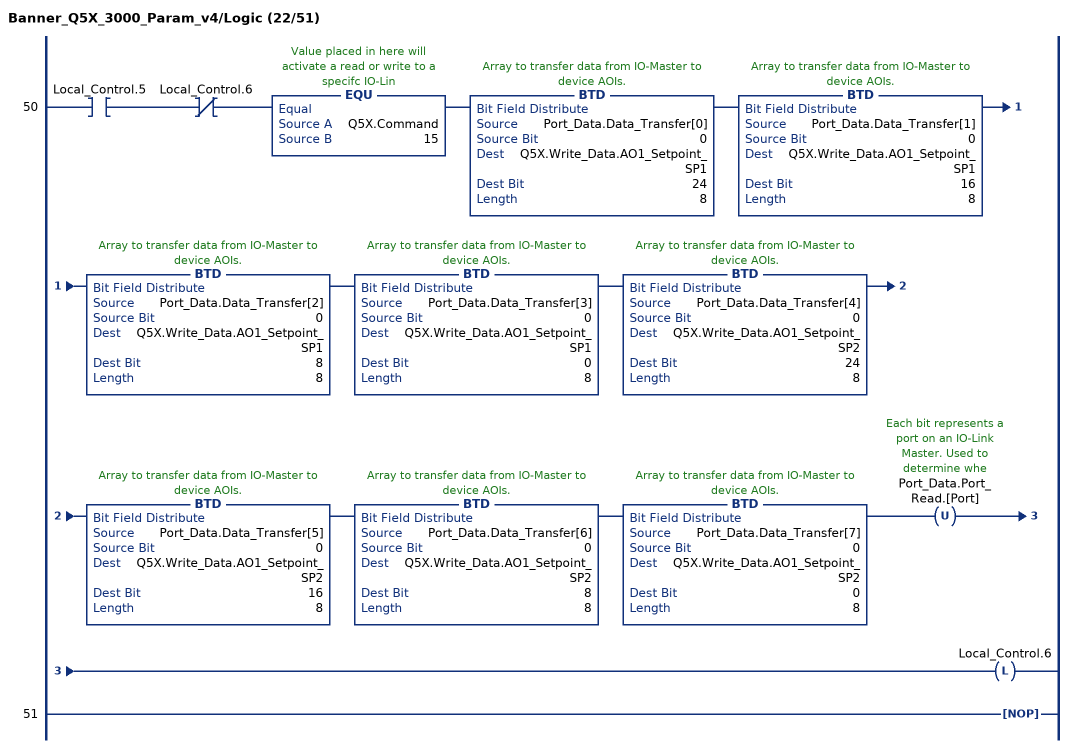
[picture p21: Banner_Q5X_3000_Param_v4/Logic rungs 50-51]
   50: XIC(Local_Control.5)XIO(Local_Control.6)EQU(Q5X.Command,15)BTD(Port_Data.Data_Transfer[0],0,Q5X.Write_Data.AO1_Setpoint_SP1,24,8)BTD(Port_Data.Data_Transfer[1],0,Q5X.Write_Data.AO1_Setpoint_SP1,16,8)BTD(Port_Data.Data_Transfer[2],0,Q5X.Write_Data.AO1_Setpoint_SP1,8,8)BTD(Port_Data.Data_Transfer[3],0,Q5X.Write_Data.AO1_Setpoint_SP1,0,8)BTD(Port_Data.Data_Transfer[4],0,Q5X.Write_Data.AO1_Setpoint_SP2,24,8)BTD(Port_Data.Data_Transfer[5],0,Q5X.Write_Data.AO1_Setpoint_SP2,16,8)BTD(Port_Data.Data_Transfer[6],0,Q5X.Write_Data.AO1_Setpoint_SP2,8,8)BTD(Port_Data.Data_Transfer[7],0,Q5X.Write_Data.AO1_Setpoint_SP2,0,8)OTU(Port_Data.Port_Read.[Port])OTL(Local_Control.6);
   51: NOP();
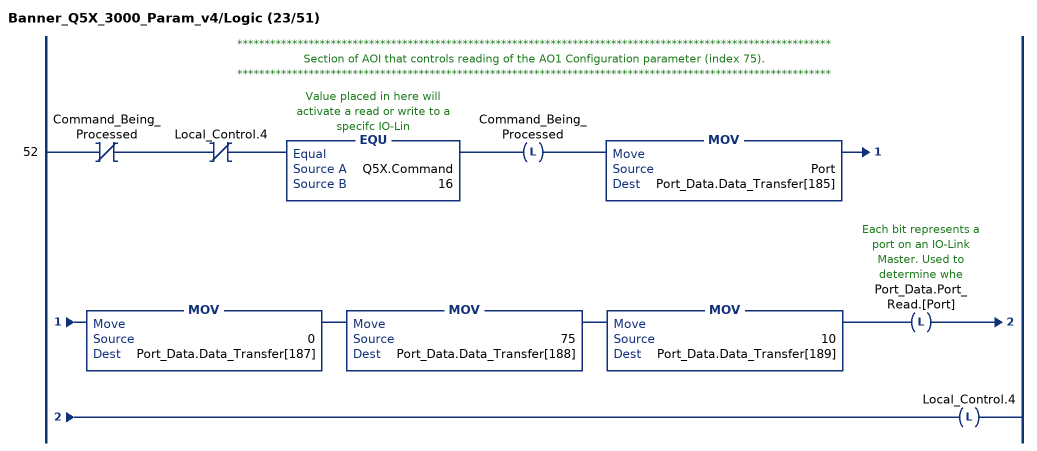
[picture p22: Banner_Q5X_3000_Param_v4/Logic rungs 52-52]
   // ************************************************************************************************************
   // Section of AOI that controls reading of the AO1 Configuration parameter (index 75).
   // ************************************************************************************************************
   52: XIO(Command_Being_Processed)XIO(Local_Control.4)EQU(Q5X.Command,16)OTL(Command_Being_Processed)MOV(Port,Port_Data.Data_Transfer[185])MOV(0,Port_Data.Data_Transfer[187])MOV(75,Port_Data.Data_Transfer[188])MOV(10,Port_Data.Data_Transfer[189])OTL(Port_Data.Port_Read.[Port])OTL(Local_Control.4);
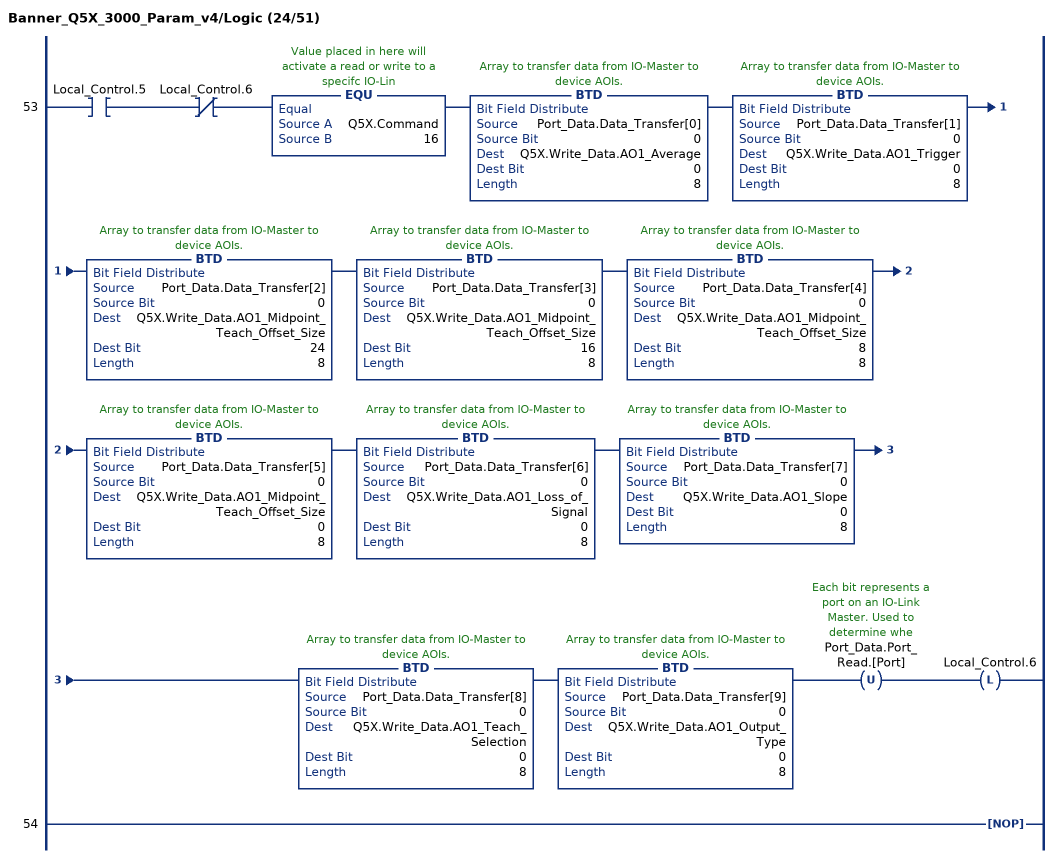
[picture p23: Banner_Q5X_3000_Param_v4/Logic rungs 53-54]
   53: XIC(Local_Control.5)XIO(Local_Control.6)EQU(Q5X.Command,16)BTD(Port_Data.Data_Transfer[0],0,Q5X.Write_Data.AO1_Average,0,8)BTD(Port_Data.Data_Transfer[1],0,Q5X.Write_Data.AO1_Trigger,0,8)BTD(Port_Data.Data_Transfer[2],0,Q5X.Write_Data.AO1_Midpoint_Teach_Offset_Size,24,8)BTD(Port_Data.Data_Transfer[3],0,Q5X.Write_Data.AO1_Midpoint_Teach_Offset_Size,16,8)BTD(Port_Data.Data_Transfer[4],0,Q5X.Write_Data.AO1_Midpoint_Teach_Offset_Size,8,8)BTD(Port_Data.Data_Transfer[5],0,Q5X.Write_Data.AO1_Midpoint_Teach_Offset_Size,0,8)BTD(Port_Data.Data_Transfer[6],0,Q5X.Write_Data.AO1_Loss_of_Signal,0,8)BTD(Port_Data.Data_Transfer[7],0,Q5X.Write_Data.AO1_Slope,0,8)BTD(Port_Data.Data_Transfer[8],0,Q5X.Write_Data.AO1_Teach_Selection,0,8)BTD(Port_Data.Data_Transfer[9],0,Q5X.Write_Data.AO1_Output_Type,0,8)OTU(Port_Data.Port_Read.[Port])OTL(Local_Control.6);
   54: NOP();
